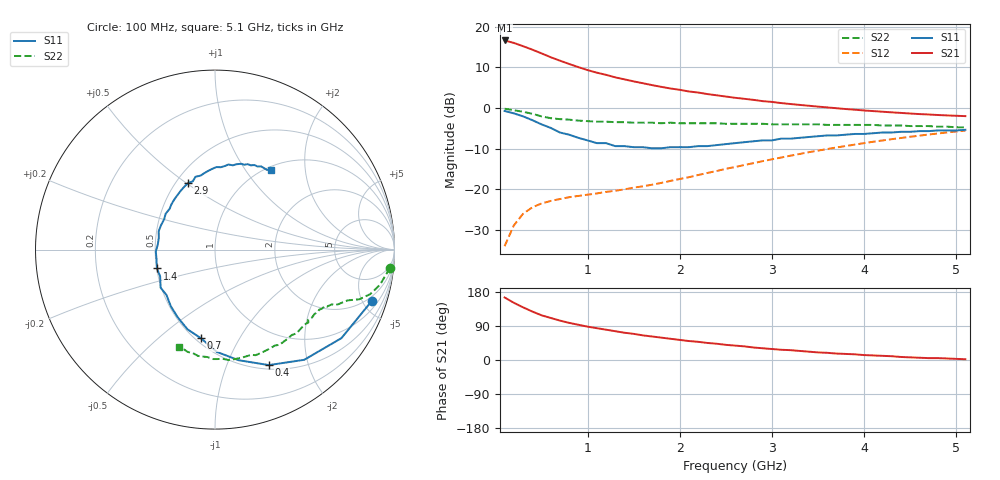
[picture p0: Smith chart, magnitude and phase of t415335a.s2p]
!AT-41533
!S and NOISE PARAMETERS at Vce=5V Ic=2mA. LAST UPDATED 01-25-95
# ghz s ma r 50
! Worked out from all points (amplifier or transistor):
!   51 points, 100 MHz to 5.1 GHz, reference 50 ohm
!   highest |S21| = 16.6 dB at 100 MHz (marker M1)
!   |S21| within 3 dB of that: start of sweep to 481.4 MHz
!   unconditionally stable (mu >= 1): 1.275 GHz to 2.197 GHz
!   at 900 MHz: K = 0.82, MSG = 15.8 dB, |S12| = -21.6 dB
!   at 2.6 GHz: K = 0.94, MSG = 8.5 dB, |S12| = -14.5 dB
!   at 5.1 GHz: K = 0.81, MSG = 1.8 dB, |S12| = -5.5 dB
!   lowest NFmin = 0.70 dB at 100 MHz
!   S11 on the Smith chart (normalised r, x): 100 MHz: 1.59, -5.89; 400 MHz: 0.55, -1.42; 700 MHz: 0.53, -0.70; 1.4 GHz: 0.50, -0.12; 2.9 GHz: 0.58, +0.51; 5.1 GHz: 1.05, +1.32
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0.1  0.92 -18.0  6.778 165.0  0.02 80.0  0.98 -6.0
0.2  0.86 -35.0  6.323 151.0  0.036 71.0  0.94 -12.0
0.3  0.79 -51.0  5.765 139.0  0.05 64.0  0.9 -16.0
0.4  0.71 -65.0  5.229 128.0  0.06 58.0  0.85 -19.0
0.5  0.63 -78.0  4.705 118.0  0.067 54.0  0.79 -21.0
0.6  0.57 -89.0  4.216 111.0  0.072 51.0  0.75 -24.0
0.7  0.5 -99.0  3.826 104.0  0.076 50.0  0.73 -25.0
0.8  0.47 -109.0  3.483 98.0  0.08 50.0  0.72 -25.0
0.9  0.43 -119.0  3.185 93.0  0.083 50.0  0.7 -27.0
1  0.4 -128.0  2.929 88.0  0.086 50.0  0.69 -27.0
1.2  0.37 -145.0  2.561 80.0  0.093 53.0  0.68 -29.0
1.3  0.34 -154.0  2.385 76.0  0.096 54.0  0.67 -30.0
1.4  0.34 -162.0  2.252 72.0  0.1 56.0  0.67 -31.0
1.6  0.33 -178.0  2.019 65.0  0.109 59.0  0.66 -34.0
1.8  0.32 168.0  1.821 59.0  0.12 62.0  0.65 -37.0
2.1  0.33 149.0  1.598 50.0  0.141 66.0  0.65 -41.0
2.6  0.37 124.0  1.337 38.0  0.188 68.0  0.64 -50.0
2.9  0.4 112.0  1.216 31.0  0.222 68.0  0.64 -56.0
3.5  0.45 92.0  1.041 20.0  0.299 63.0  0.63 -69.0
4  0.48 78.0  0.933 13.0  0.37 58.0  0.62 -81.0
4.3  0.5 71.0  0.885 10.0  0.414 53.0  0.61 -89.0
5.1  0.54 55.0  0.795 2.0  0.528 41.0  0.58 -110.0
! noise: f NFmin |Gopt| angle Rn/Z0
0.1  0.7  0.56  7  0.26
0.9  1.1  0.35  78  0.2
1.8  1.6  0.39  155  0.11
2.4  2.1  0.52  195  0.09
